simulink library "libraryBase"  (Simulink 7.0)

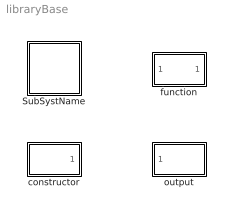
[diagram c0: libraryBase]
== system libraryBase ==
  SubSystName : Subsystem  Tag=subsystem
  constructor : Subsystem  Tag=subsystem
  function : Subsystem  Tag=subsystem
  output : Subsystem  Tag=subsystem

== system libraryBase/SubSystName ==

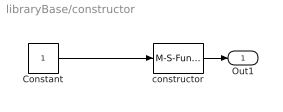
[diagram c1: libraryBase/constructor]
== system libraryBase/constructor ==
  Constant : Constant  OutDataType=sfix(16)  OutScaling=2^0
  constructor : M-S-Function  Tag=function  FunctionName=ltpdasim
  Out1 : Outport  OutDataType=sfix(16)  OutScaling=2^0
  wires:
  constructor/1 -> Out1/1
  Constant/1 -> constructor/1

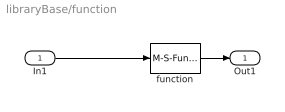
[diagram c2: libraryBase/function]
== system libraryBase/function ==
  In1 : Inport  OutDataType=sfix(16)  OutScaling=2^0
  function : M-S-Function  Tag=function  FunctionName=ltpdasim
  Out1 : Outport  OutDataType=sfix(16)  OutScaling=2^0
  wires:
  function/1 -> Out1/1
  In1/1 -> function/1

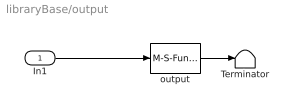
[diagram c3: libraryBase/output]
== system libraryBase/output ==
  In1 : Inport  OutDataType=sfix(16)  OutScaling=2^0
  Terminator : Terminator
  output : M-S-Function  Tag=function  FunctionName=ltpdasim
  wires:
  In1/1 -> output/1
  output/1 -> Terminator/1
